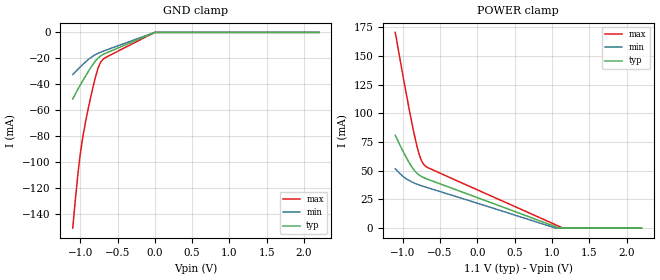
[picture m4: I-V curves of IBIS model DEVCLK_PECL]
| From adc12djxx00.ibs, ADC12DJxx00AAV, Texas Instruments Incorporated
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|   Model DEVCLK
[Model]   DEVCLK_PECL
Model_type   Input
Vinl = .57
Vinh = 1.33
|   typ   min   max
|   (nom PVT)   (slow PVT)   (fast PVT)
C_comp   1.800p   1.766p   1.839p
[Voltage Range]   1.1   1.05   1.15
[Temperature Range]   27   125   -40
[Power Clamp Reference]   1.1   1.05   1.15
[GND Clamp Reference]   0   0   0
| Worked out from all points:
|   GND clamp passes 1 mA (typ) near -0.04 V on its own axis
[GND Clamp]
|   Voltage   I(typ)   I(min)   I(max)
-1.1V     -51.31mA   -32.47mA   -150.9mA
-1.064V   -47.26mA   -30.32mA   -128mA
-1.031V   -43.8mA    -28.4mA    -109.1mA
-1.008V   -41.44mA   -27.09mA   -97.55mA
-971.3mV  -37.8mA    -25.06mA   -82.65mA
-928.4mV  -33.61mA   -22.78mA   -68.92mA
-812.9mV  -23.35mA   -17.68mA   -38.28mA
-763.4mV  -19.97mA   -16.18mA   -28.05mA
-723.8mV  -18.07mA   -15.21mA   -22.78mA
-680.9mV  -16.66mA   -14.26mA   -20.1mA
-1.1mV    -27.02uA   -23.17uA   -32.95uA
2.2V      0A         0A         0A
[POWER Clamp]
|   Voltage   I(typ)   I(min)   I(max)
-1.1V     80.89mA    51.71mA    170.6mA
-997.7mV  67.25mA    45.15mA    133.2mA
-925.1mV  58.37mA    41.92mA    107.7mA
-836mV    49.72mA    39.01mA    78.91mA
-796.4mV  47.18mA    37.99mA    68.17mA
-753.5mV  45.2mA     37.03mA    59.56mA
-717.2mV  43.96mA    36.27mA    55.42mA
-697.4mV  43.39mA    35.87mA    54.12mA
1.048V    1.255mA    35.29uA    2.961mA
1.098V    53.14uA    0A         1.519mA
1.147V    0A         0A         77.72uA
2.2V      0A         0A         0A
